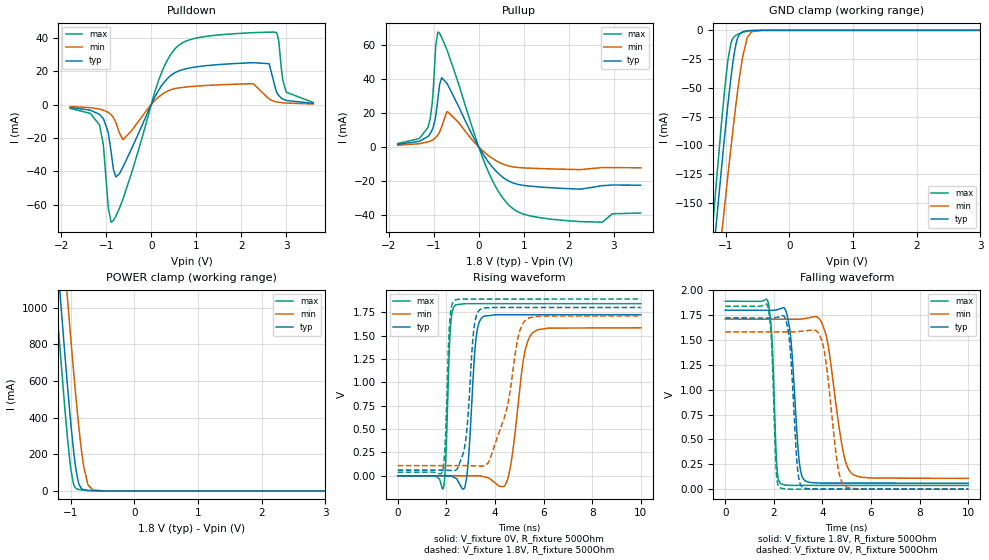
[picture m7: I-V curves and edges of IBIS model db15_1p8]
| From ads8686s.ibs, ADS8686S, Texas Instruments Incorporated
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|   db15_1p8 Model
[Model]   db15_1p8
Model_type   I/O
Polarity   Non-Inverting
Enable   Active-Low
Vinl = 0.54
Vinh = 1.26
Vmeas = 0.9
Vref = 0.9
Cref = 15pF
Rref = 50
|   typ   min   max
C_comp   1.54pF   1.54pF   1.57pF
[Voltage Range]   1.8   1.71   1.89
[Temperature Range]   27   125   -40
[Pullup Reference]   1.8   1.71   1.89
[Pulldown Reference]   -0   0   0
[Power Clamp Reference]   1.8   1.71   1.89
[GND Clamp Reference]   0   0   0
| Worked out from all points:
|   slope of the pulldown table from 0 to 0.27 V, typ, clamps not added: 21 ohm
|   slope of the pullup table from 0 to 0.27 V, typ, clamps not added: 25.2 ohm
|   GND clamp passes 1 mA (typ) near -0.72 V on its own axis
|   POWER clamp passes 1 mA (typ) near -0.62 V on its own axis
|   falling waveform, V_fixture 1.8V, R_fixture 500Ohm: 20-80 % time 275ps typ, 540ps min, 166ps max; typ from 1.8 V to 0.06 V
|   rising waveform, V_fixture 0V, R_fixture 500Ohm: 20-80 % time 233ps typ, 428ps min, 140ps max; typ from 0 V to 1.72 V
|   rising waveform, V_fixture 1.8V, R_fixture 500Ohm: 20-80 % time 278ps typ, 760ps min, 148ps max; typ from 0.06 V to 1.8 V
|   falling waveform, V_fixture 0V, R_fixture 500Ohm: 20-80 % time 246ps typ, 429ps min, 157ps max; typ from 1.72 V to 0 V
[Pulldown]
|   Voltage   I(typ)   I(min)   I(max)
-1.8V     -1.668mA   -1.055mA   -2.244mA
-1.152V   -5.773mA   -2.622mA   -12.03mA
-1.066V   -8.32mA    -3.247mA   -23.76mA
-887.4mV  -29.12mA   -6.096mA   -70.63mA
-709.2mV  -41.62mA   -16.82mA   -62.49mA
230.4mV   11.41mA    6.006mA    19.3mA
689.4mV   20.98mA    10.36mA    37.1mA
2.266V    25.24mA    12.61mA    43.3mA
2.617V    24.64mA    3.483mA    43.58mA
2.768V    8.842mA    1.774mA    43.4mA
3.001V    2.503mA    964.9uA    7.472mA
3.6V      800.2uA    430.1uA    1.306mA
[GND Clamp]
|   Voltage   I(typ)   I(min)   I(max)
-1.8V     -575.1mA   -590.1mA   -589.5mA
-1.211V   -205.2mA   -256.8mA   -174.1mA
-1.152V   -169.4mA   -224.2mA   -134.4mA
-1.066V   -118.7mA   -177.6mA   -79.19mA
-1.017V   -91.27mA   -151.8mA   -50.81mA
-963mV    -62.4mA    -123.9mA   -24.53mA
-903.6mV  -34.11mA   -94.13mA   -8.664mA
-822.6mV  -8.191mA   -56.42mA   -3.809mA
-736.2mV  -1.24mA    -23.24mA   -1.747mA
-666mV    -402uA     -6.834mA   -720.4uA
-595.8mV  -133uA     -1.235mA   -229.3uA
3.6V      0A         0A         0A
[Pullup]
|   Voltage   I(typ)   I(min)   I(max)
-1.8V     1.542mA    1.017mA    2.04mA
-1.336V   3.252mA    1.88mA     4.844mA
-1.13V    6.161mA    2.965mA    11.47mA
-1.039V   9.826mA    3.95mA     24.5mA
-952.2mV  18.85mA    5.621mA    60.35mA
-903.6mV  29.12mA    7.211mA    67.66mA
-822.6mV  40.83mA    11.98mA    64.46mA
-693mV    36.85mA    20.85mA    56.33mA
144mV     -6.171mA   -3.541mA   -10.24mA
689.4mV   -20.34mA   -11.32mA   -34.72mA
2.261V    -24.83mA   -13.29mA   -43.94mA
3.6V      -22.51mA   -12.26mA   -38.89mA
[POWER Clamp]
|   Voltage   I(typ)   I(min)   I(max)
-1.8V     4.061A     4.54A      3.768A
-1.233V   1.367A     1.858A     1.061A
-1.179V   1.123A     1.613A     817.9mA
-1.049V   564.5mA    1.04A      280.1mA
-995.4mV  355.2mA    812.6mA    109.9mA
-963mV    243.1mA    681mA      46.78mA
-914.4mV  108.2mA    493.5mA    12.79mA
-865.8mV  32.73mA    323.4mA    7.075mA
-795.6mV  5.598mA    130.2mA    4.664mA
-730.8mV  2.41mA     35.35mA    3.08mA
-649.8mV  1.154mA    4.788mA    1.533mA
3.6V      0A         0A         0A
[Ramp]
R_load = 500
|   typ   min   max
dV/dt_r   1.03354/2.32588e-10   0.949545/4.27148e-10   1.10446/1.39975e-10
dV/dt_f   1.0439/2.7456e-10   0.960922/5.39602e-10   1.11143/1.66116e-10
[Falling Waveform]
V_fixture = 1.8V
V_fixture_min = 1.71V
V_fixture_max = 1.89V
R_fixture = 500Ohm
C_fixture = 0F
|   Time   V(typ)   V(min)   V(max)
0s        1.8V       1.71V      1.89V
1.742ns   1.799V     1.709V     1.898V
2.127ns   1.804V     1.709V     218.5mV
2.28ns    1.816V     1.709V     56.2mV
2.649ns   1.615V     1.709V     39.12mV
3.038ns   295.8mV    1.71V      37.89mV
3.283ns   84.76mV    1.716V     37.88mV
4.087ns   60.91mV    1.599V     37.85mV
5.249ns   60.76mV    149.3mV    37.8mV
10ns      60.17mV    108.5mV    37.61mV
[Rising Waveform]
V_fixture = 0V
V_fixture_min = 0V
V_fixture_max = 0V
R_fixture = 500Ohm
C_fixture = 0F
|   Time   V(typ)   V(min)   V(max)
0s        -31nV      2.475uV    -37.3nV
1.874ns   -644.1uV   -212uV     -136.4mV
2.166ns   -744.6uV   -245.5uV   1.57V
2.376ns   -25.49mV   -269.5uV   1.826V
2.827ns   -39.7mV    -321.2uV   1.841V
3.223ns   1.469V     -366.4uV   1.841V
3.518ns   1.703V     -9.171mV   1.841V
4.509ns   1.722V     -48.23mV   1.841V
5.546ns   1.722V     1.527V     1.841V
10ns      1.723V     1.583V     1.841V
[Rising Waveform]
V_fixture = 1.8V
V_fixture_min = 1.71V
V_fixture_max = 1.89V
R_fixture = 500Ohm
C_fixture = 0F
|   Time   V(typ)   V(min)   V(max)
0s        60.17mV    108.5mV    37.61mV
1.835ns   60.95mV    108.7mV    42.51mV
2.141ns   57.21mV    108.8mV    1.654V
2.331ns   54.29mV    108.8mV    1.875V
2.789ns   363.2mV    108.9mV    1.89V
3.123ns   1.544V     106.1mV    1.89V
3.392ns   1.779V     102.7mV    1.89V
4.379ns   1.8V       615.1mV    1.89V
5.21ns    1.8V       1.651V     1.89V
10ns      1.8V       1.71V      1.89V
[Falling Waveform]
|Gnd
V_fixture = 0V
V_fixture_min = 0V
V_fixture_max = 0V
R_fixture = 500Ohm
C_fixture = 0F
|   Time   V(typ)   V(min)   V(max)
0s        1.723V     1.583V     1.841V
1.742ns   1.722V     1.582V     1.846V
2.103ns   1.726V     1.582V     169.4mV
2.238ns   1.736V     1.582V     17.03mV
2.629ns   1.52V      1.582V     887.7uV
2.979ns   198.5mV    1.584V     304.1uV
3.187ns   18.39mV    1.59V      295.1uV
4.012ns   576.4uV    1.458V     259.4uV
4.95ns    486.1uV    26.27mV    218.8uV
10ns      171.4nV    2.069uV    18.32nV
